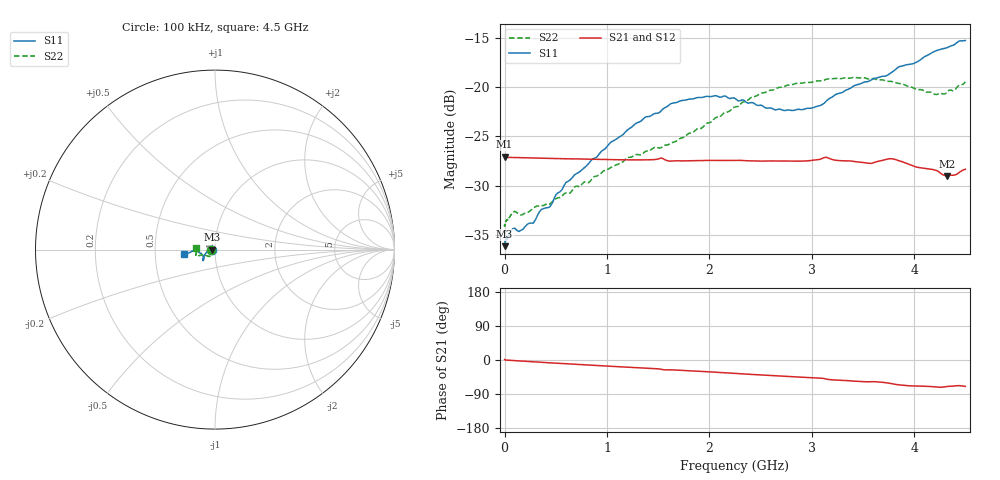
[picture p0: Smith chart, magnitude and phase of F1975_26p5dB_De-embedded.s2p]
! Integrated Device Technology
! Corporate Headquarters
! 6024 Silver Creek Valley Road
! San Jose, CA 95138  USA
! Phone:  1-408-284-8200
! Toll Free:  1-800-223-1366
! Webpage:  http://www.idt.com/
! Timing and RF Division
! 515 Groton Road, Suite 102
! Westford, MA 01886-6024
! Device:  F1975
! Description: 6-bit, 75 ohm, 0.5 dB Digital Step Attenuator
! Frequency:  5.0 MHz -  3.00 GHz
! Package:  4x4 mm QFN Plastic Package: 20 pin
! Ports:  2 RF, 11 DC
!  Pin  1  = D5 (16 dB)
!  Pin  2  = RF1  =  Port 1
!  Pin  3  = Serial Data In (DATA)
!  Pin  4  = Serial Clock (CLK)
!  Pin  5  = Serial Latch Enable (LE)
!  Pin  6  = VDD
!  Pin  7  = NC
!  Pin  8  = NC
!  Pin  9  = NC
!  Pin 10  = GND
!  Pin 11  = GND
!  Pin 12  = NC
!  Pin 13  = VMODE
!  Pin 14  = RF2  =  Port 2
!  Pin 15  = D4 (8 dB)
!  Pin 16  = D3 (4 dB)
!  Pin 17  = D2 (2 dB)
!  Pin 18  = NC
!  Pin 19  = D1 (1 dB)
!  Pin 20  = D0 (0.5 dB)
! State:  53
! Atten State:  26.5 dB
! Voltage:  +3.30 Volts
! Current:  0.561 mA
! Data:  The device was measured on a F1975 evaluation board which has
!  individual transmission lines to the RF pins.  Data was collected
!  using a calibrated network analyzer.  The evaluation board was
!  de-embedded using Automatic Fixture Removal (AFR).
!  The reference plane is the edge of the package pin.
! Misc:
!  Action Tracker AT0415
! Date Measured:  2018-02-08
! Date:  2018-03-26  MJV
! Note:
!  Integrated Device Technology supplies this data as a sample of measured
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# GHz S dB R 75
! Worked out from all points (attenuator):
!   291 points, 100 kHz to 4.5 GHz, reference 75 ohm
!   highest |S21| = -27.04 dB at 100 kHz (marker M1); lowest = -29.0 dB at 4.32 GHz (marker M2)
!   lowest |S11| = -36.1 dB at 100 kHz (marker M3), VSWR 1.03, Z = 72.7 - j0.00375 ohm
!   |S11| at or under -10 dB: start of sweep to end of sweep
!   |S22| runs from -34.1 to -19.0 dB; largest |S21 - S12| = 0.00017
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0.0001  -36.10 -179.9  -27.04 1.2  -27.07 1.2  -34.08 -179.1
0.007  -35.57 -178.1  -27.10 0.2  -27.12 0.1  -33.66 -177.2
0.08  -34.33 -176.4  -27.13 -1.5  -27.12 -1.4  -32.67 -169.0
0.14  -34.62 -175.6  -27.14 -2.5  -27.14 -2.5  -32.83 -160.4
0.28  -33.78 180.0  -27.18 -4.8  -27.17 -4.8  -32.26 -151.4
0.36  -32.38 180.0  -27.20 -6.1  -27.20 -6.1  -32.00 -143.7
0.44  -32.13 -179.4  -27.21 -7.4  -27.21 -7.4  -31.87 -137.7
0.6  -29.65 -175.9  -27.26 -9.9  -27.25 -9.9  -30.70 -131.8
0.76  -28.33 -169.4  -27.29 -12.3  -27.29 -12.3  -29.78 -128.0
1.28  -23.69 -152.8  -27.37 -20.1  -27.37 -20.1  -26.84 -123.9
1.52  -22.51 -144.8  -27.21 -23.9  -27.21 -23.9  -26.17 -130.6
1.62  -21.70 -143.1  -27.50 -26.0  -27.49 -26.0  -25.71 -134.1
1.88  -21.07 -139.0  -27.45 -29.3  -27.45 -29.3  -24.24 -146.6
2.26  -21.23 -138.0  -27.43 -35.5  -27.42 -35.5  -21.99 -157.7
2.64  -22.31 -147.4  -27.48 -41.5  -27.48 -41.5  -20.24 -159.2
3.02  -22.07 -163.7  -27.39 -47.0  -27.39 -47.0  -19.45 -159.9
3.14  -21.43 -166.7  -27.10 -50.3  -27.10 -50.3  -19.22 -160.4
3.58  -19.29 -177.2  -27.73 -57.3  -27.73 -57.3  -19.17 -166.4
3.76  -18.66 -175.8  -27.25 -61.4  -27.25 -61.4  -19.43 -169.7
4.2  -16.39 -172.7  -28.40 -70.9  -28.39 -70.9  -20.74 178.8
4.32  -16.02 -172.4  -28.99 -70.0  -28.98 -70.1  -20.54 176.5
4.5  -15.29 -172.3  -28.32 -69.8  -28.31 -69.8  -19.47 173.9
